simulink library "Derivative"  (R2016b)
settings: Solver=VariableStepAuto  StartTime=0.0  StopTime=10.0  RelTol=1e-3
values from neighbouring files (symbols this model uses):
  a = ( ax.^2 + ay.^2 + az.^2 ).^0.5    [microcart_imu_analysis_1.m]
undefined symbols (not defined in the file or in its folder): Ts
libraries: simulink x1

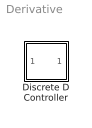
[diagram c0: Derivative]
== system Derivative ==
  Discrete D Controller : Subsystem  TreatAsAtomicUnit=on  SystemSampleTime=Ts

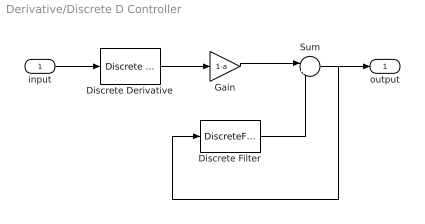
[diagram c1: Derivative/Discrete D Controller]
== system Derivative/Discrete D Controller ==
  input : Inport
  Discrete Derivative : simulink/Discrete/Discrete Derivative  gainval=Kd  ICPrevScaledInput=0.0  OutMin=[]  OutMax=[]  OutDataType=fixdt(1, 16)  OutScaling=2^-10  DoSatur=off
  Discrete Filter : DiscreteFilter  Numerator=[0 a]  Denominator=[1]
  Gain : Gain  Gain=1-a
  Sum : Sum  Inputs=|++
  output : Outport
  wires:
  Discrete Derivative/1 -> Gain/1
  Discrete Filter/1 -> Sum/2
  Sum/1 -> output/1, Discrete Filter/1
  input/1 -> Discrete Derivative/1
  Gain/1 -> Sum/1
